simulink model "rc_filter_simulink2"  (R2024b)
settings: Solver=VariableStepAuto  StartTime=0.0  StopTime=10.0  RelTol=1e-3
libraries: simulink x2

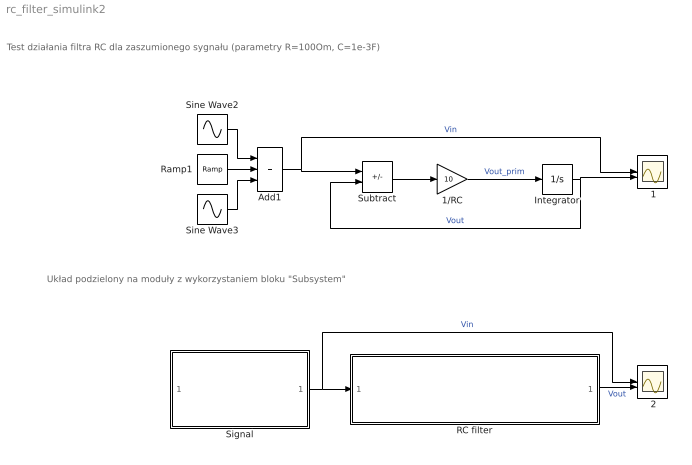
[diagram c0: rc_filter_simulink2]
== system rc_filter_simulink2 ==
  note: Test działania filtra RC dla zaszumionego sygnału (parametry R=100Om, C=1e-3F)
  note: Układ podzielony na moduły z wykorzystaniem bloku "Subsystem"
  " 1" : Scope  NumInputPorts=2
  " 2" : Scope  NumInputPorts=2
  1/RC : Gain  Gain=10
  Add1 : Sum  Inputs=+++
  Integrator : Integrator
  RC filter : Subsystem
  Ramp1 : simulink/Sources/Ramp  slope=0.25  start=0  InitialOutput=0
  Signal : Subsystem
  Sine Wave2 : Sin  Amplitude=2  Frequency=1.57  SampleTime=0
  Sine Wave3 : Sin  Amplitude=0.1  Frequency=31  SampleTime=0
  Subtract : Sum  Inputs=+-
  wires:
  1/RC/1 -> Integrator/1  "Vout_prim"
  Integrator/1 -> Subtract/2, " 1"/2  "Vout"
  Add1/1 -> Subtract/1, " 1"/1  "Vin"
  Subtract/1 -> 1/RC/1
  Ramp1/1 -> Add1/2
  Sine Wave3/1 -> Add1/3
  Sine Wave2/1 -> Add1/1
  Signal/1(Vin) -> " 2"/1, RC filter/1(Vin)  "Vin"
  RC filter/1(Vout) -> " 2"/2  "Vout"

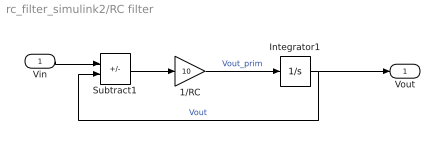
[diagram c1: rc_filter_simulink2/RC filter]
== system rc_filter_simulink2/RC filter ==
  Vin : Inport
  1/RC : Gain  Gain=10
  Integrator1 : Integrator
  Subtract1 : Sum  Inputs=+-
  Vout : Outport
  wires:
  Vin/1 -> Subtract1/1
  Subtract1/1 -> 1/RC/1
  Integrator1/1 -> Vout/1, Subtract1/2  "Vout"
  1/RC/1 -> Integrator1/1  "Vout_prim"

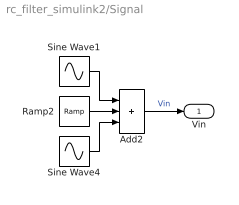
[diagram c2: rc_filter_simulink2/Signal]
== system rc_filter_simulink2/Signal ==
  Add2 : Sum  Inputs=+++
  Ramp2 : simulink/Sources/Ramp  slope=0.25  start=0  InitialOutput=0
  Sine Wave1 : Sin  Amplitude=2  Frequency=1.57  SampleTime=0
  Sine Wave4 : Sin  Amplitude=0.1  Frequency=31  SampleTime=0
  Vin : Outport
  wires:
  Ramp2/1 -> Add2/2
  Sine Wave1/1 -> Add2/1
  Add2/1 -> Vin/1  "Vin"
  Sine Wave4/1 -> Add2/3
